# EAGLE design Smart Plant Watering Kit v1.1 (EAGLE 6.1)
COMPANY: ADAFRUIT INDUSTRIES; DRAWN: KTOWN; REV: B
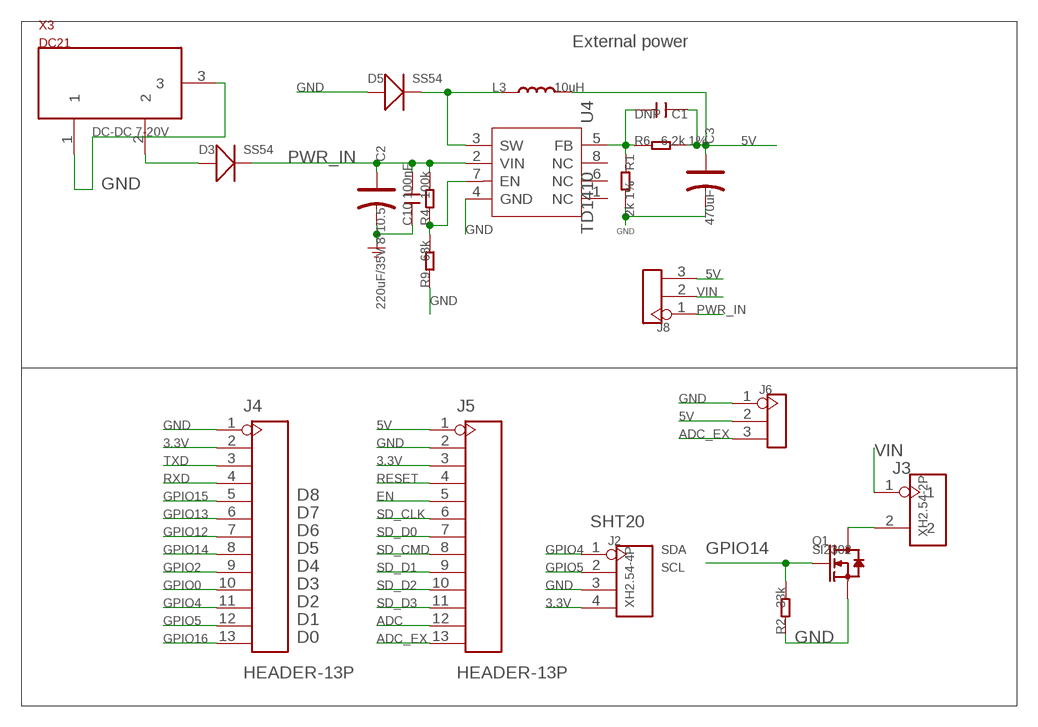
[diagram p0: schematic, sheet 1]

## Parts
C1  DNP  C-0603  [C0603]
C2  220uF/35V 8*10.5  CAP-ELECTRO-E  [ELECTRO-SMD-E-7.8MM]
C3  470uF  CAP-AVX-D  [AVX-D]
C10  100nF  C-0603  [C0603]
D3  SS54  D'SMA'  [D2010]
D5  SS54  D'SMA'  [D2010]
J2  XH2.54-4P  [XH2.54-4P]
J3  XH2.54-2P  [XH2.54-2P]
J4  HEADER-13P  [13P-2.54]
J5  HEADER-13P  [13P-2.54]
J6  HEADER-3P-2.54  [3P-2.54]
J8  HEADER-3P-2.54  [3P-2.54]
L3  10uH  DISCRETE_L0630  [L0630]
Q1  SI2302  MOSFET-N'SOT23'  [SOT23]
R1  2k 1%  R-0603  [R0603]
R2  33k  R-0603  [R0603]
R4  100k  R-0603  [R0603]
R6  6.2k 1%  R-0603  [R0603]
R9  68k  R-0603  [R0603]
U4  TD1410  [SOP8]
X3  DC21  POWERSUPPLY_DC21MMX  [POWERSUPPLY_DC-21MM]

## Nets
3.3V: J2.4 J4.2 J5.3
5V: C1.1 C3.+ J5.1 J6.2 J8.3 L3.2 R6.2
ADC: J5.12
ADC_EX: J5.13 J6.3
EN: J5.5
GND: C2.- C3.- C10.1 D5.+ J2.3 J4.1 J5.2 J6.1 Q1.2(S) R1.2 R2.1 R9.1 U4.4(GND) X3.1 X3.3
GPIO0: J4.10
GPIO2: J4.9
GPIO4: J2.1 J4.11
GPIO5: J2.2 J4.12
GPIO12: J4.7
GPIO13: J4.6
GPIO14: J4.8 Q1.1(G) R2.2
GPIO15: J4.5
GPIO16: J4.13
N$1: D3.+ X3.2
N$4: J3.2 Q1.3(D)
N$12: R4.1 R9.2 U4.7(EN)
N$38: D5.- L3.1 U4.3(SW)
N$47: C1.2 R1.1 R6.1 U4.5(FB)
PWR_IN: C2.+ C10.2 D3.- J8.1 R4.2 U4.2(VIN)
RESET: J5.4
RXD: J4.4
SD_CLK: J5.6
SD_CMD: J5.8
SD_D0: J5.7
SD_D1: J5.9
SD_D2: J5.10
SD_D3: J5.11
TXD: J4.3
VIN: J3.1 J8.2
Unconnected: U4.1(NC) U4.6(NC) U4.8(NC)

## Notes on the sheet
- External power
- DC-DC 7-20V
- D8
- D7
- SHT20
- D6
- D5 | SDA
- D4 | SCL
- D3
- D2
- D1
- D0

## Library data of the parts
C1 C10 = Discrete:C*: Ceramic Capacitors
C2 C3 = Discrete:CAP*: Electrolytic Capacitors,Tantalum Capacitors and Super Capacitors
D3 D5 = Discrete:D*
J2 = Connector:XH2.54-4P
J3 = Connector:XH2.54-2P
J4 J5 = Connector:HEADER-13P
J6 J8 = Connector:HEADER-3P
L3 = L:DISCRETE_L*
Q1 = Discrete:MOSFET-N: IRLL014: http://www.vishay.com/docs/91319/sihll014.pdf
R1 R2 R4 R6 R9 = Discrete:R*
U4 = template:TD1410: 2A 380KHz 20V PWM Buck DC/DC Converter
X3 = SmartPrj:POWERSUPPLY_DC21MM

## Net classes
0 default: width 0.203 mm, drill 0.305 mm, clearance 0.152 mm

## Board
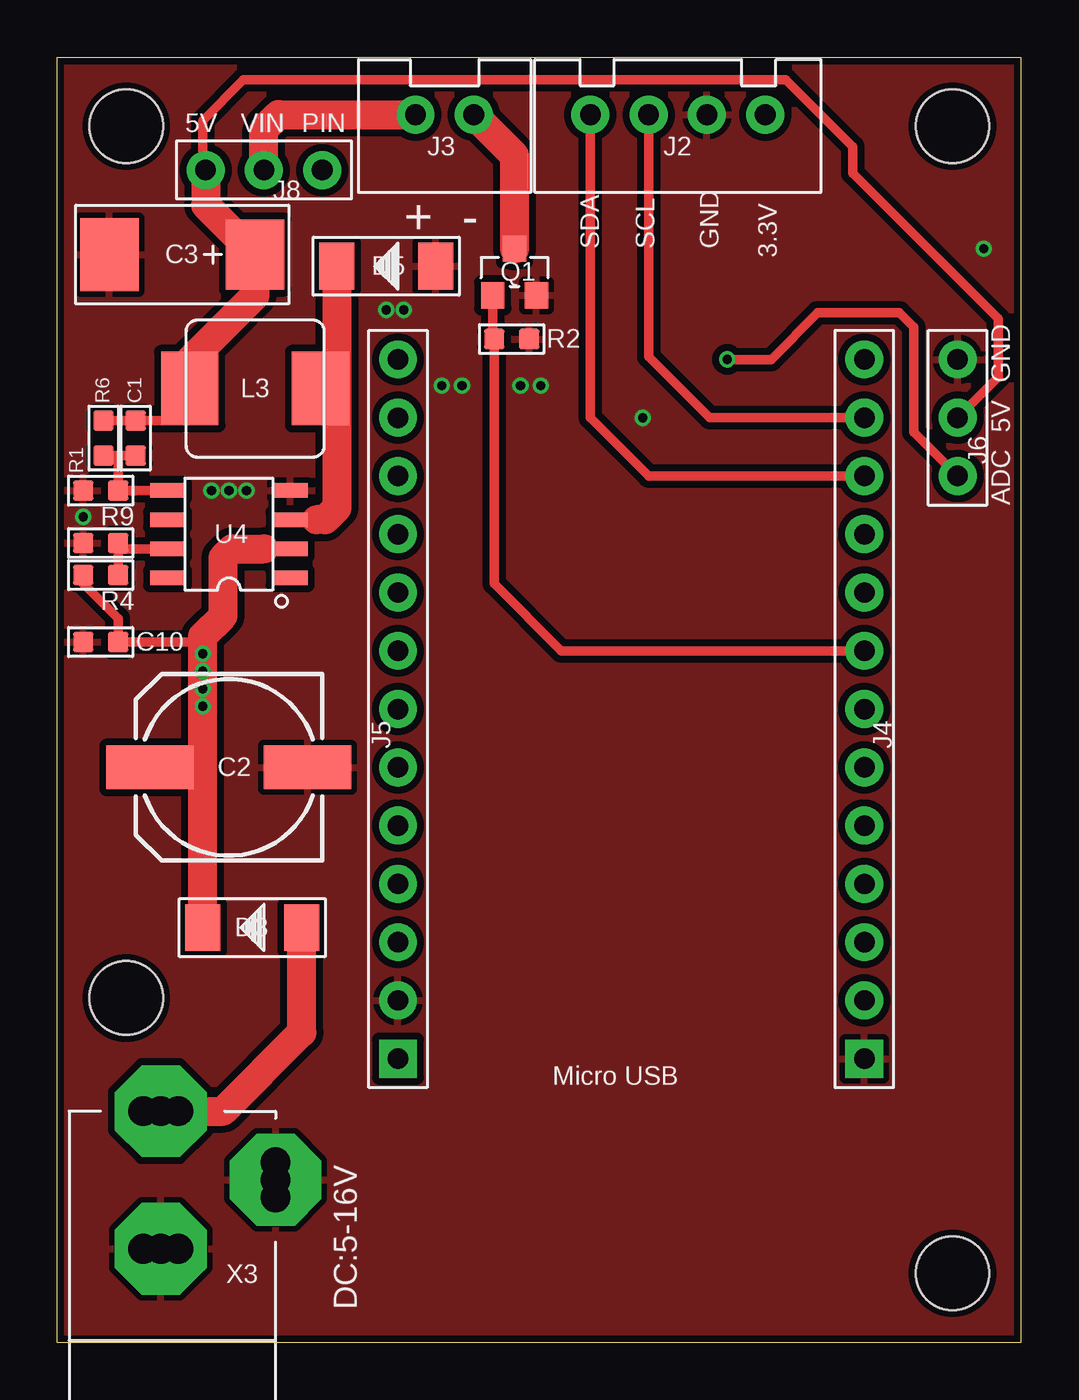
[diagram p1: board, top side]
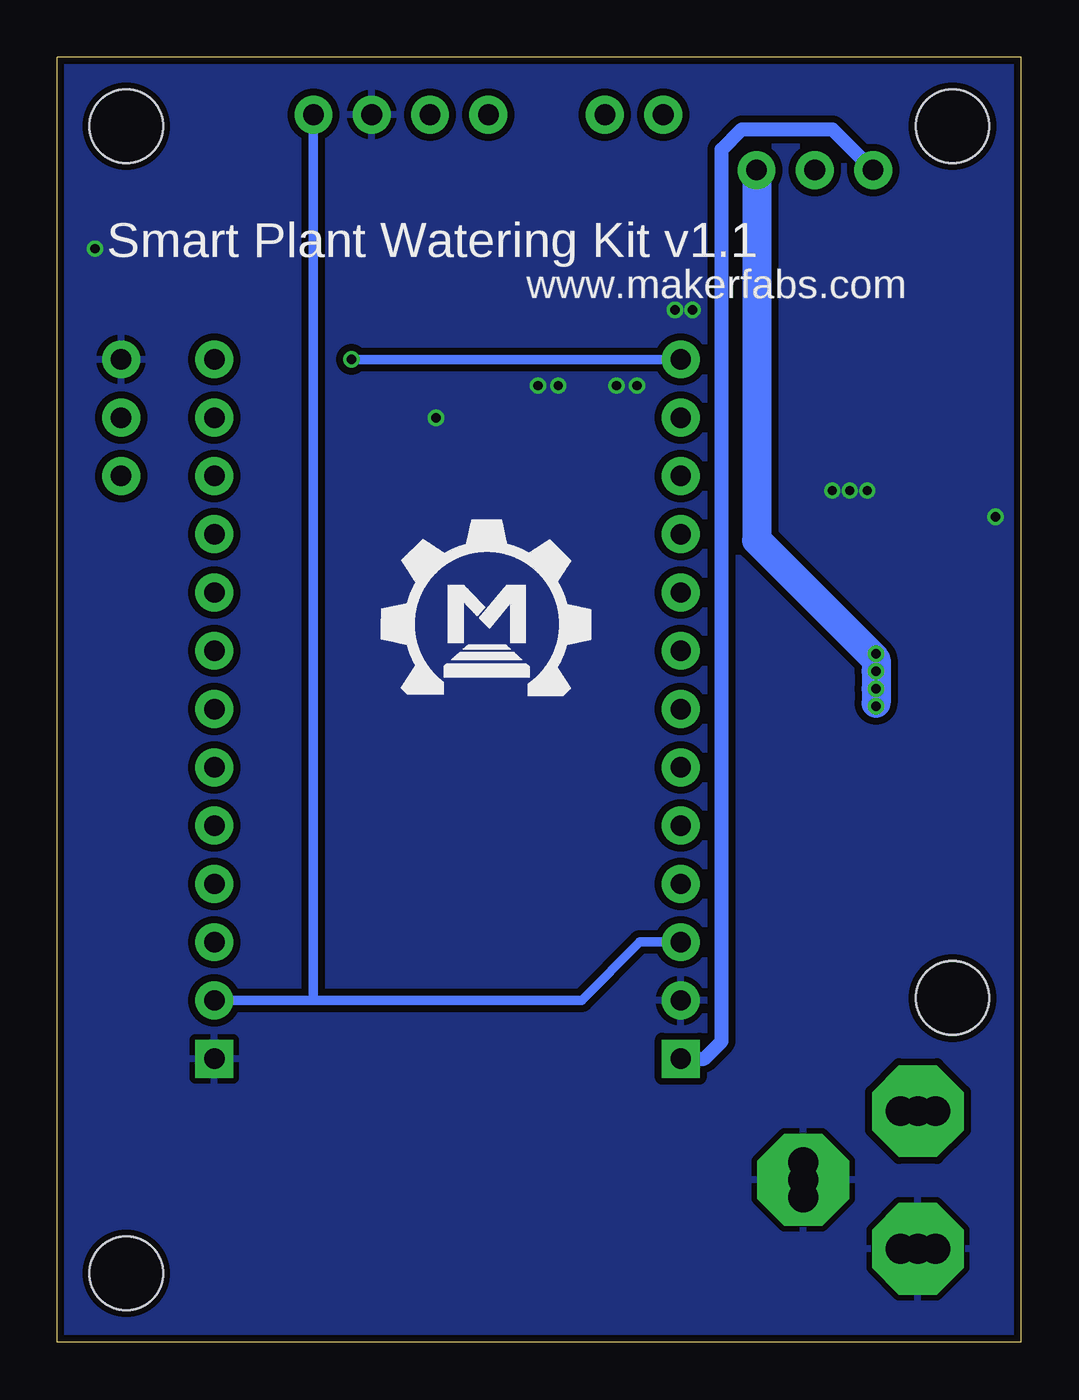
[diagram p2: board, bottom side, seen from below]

Size 42 x 56 mm. Coordinates in mm from the lower left corner, seen from the top.
Outline: 42,0 42,56 0,56 0,0 42,0
Copper layers (1*16): Top 0.035mm / dielectric 1.5mm / Bottom 0.035mm
Design rules: minimum track width 6mil, minimum drill 12mil, track to track 6mil, track to pad 6mil, pad to pad 6mil, via to via 6mil, smd to smd 0mil, copper to edge 10mil, drill to drill 10mil, minimum pad ring 10mil, minimum via ring 6mil, stop-mask expansion 2mil, vias tented up to drill 100mil, thermal gap 10mil
Holes 3.2 mm at 39,3 3,53 39,53 3,15

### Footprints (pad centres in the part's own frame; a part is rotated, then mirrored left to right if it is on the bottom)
C0603 = smd 0.889 x 0.889: 1 -0.762,0; 2 0.762,0
ELECTRO-SMD-E-7.8MM = smd 3.81 x 1.905: + 3.429,0; - -3.429,0
AVX-D = smd 2.54 x 3.048: + -3.175,0 | smd 2.54 x 3.175: - 3.175,0
D2010 = smd 1.524 x 2.032: + -2.159,0; - 2.159,0
XH2.54-4P = drill 0.9 pad 1.651: 1 -3.81,0; 2 -1.27,0; 3 1.27,0; 4 3.81,0
XH2.54-2P = drill 0.9 pad 1.651: 1 -1.27,0; 2 1.27,0
13P-2.54 = drill 0.889 pad 1.651 square: 1 0,15.24 | drill 0.889 pad 1.651: 2 0,12.7; 3 0,10.16; 4 0,7.62; 5 0,5.08; 6 0,2.54; 7 0,0; 8 0,-2.54; 9 0,-5.08; 10 0,-7.62; 11 0,-10.16; 12 0,-12.7; 13 0,-15.24
3P-2.54 = drill 0.9 pad 1.651: 1 0,2.54; 2 0,0; 3 0,-2.54
L0630 = smd 2.5 x 3.2: 1 -2.85,0; 2 2.85,0
SOT23 = smd 1.016 x 1.143: 1 -0.95,-1.016; 2 0.95,-1.016; 3 0,1.016
R0603 = smd 0.889 x 0.889: 1 -0.762,0; 2 0.762,0
SOP8 = smd 0.635 x 1.524: 1 -1.905,-2.667; 2 -0.635,-2.667; 3 0.635,-2.667; 4 1.905,-2.667; 5 1.905,2.667; 6 0.635,2.667; 7 -0.635,2.667; 8 -1.905,2.667
POWERSUPPLY_DC-21MM = drill 1.3 pad 4 octagon: 1 -5.08,-3.353; 2 -0.076,-6.35; 3 -0.076,-0.356 | drill 1.3: 4 -5.08,-4.115; 5 -5.08,-2.591; 6 -0.838,-0.356; 7 0.686,-0.356; 8 -0.838,-6.35; 9 0.686,-6.35

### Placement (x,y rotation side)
C1  3.41,39.41 270 top
C2  7.47,25.05 180 top
C3  5.44,47.41 180 top
C10  1.89,30.52 0 top
D3  8.49,18.07 180 top
D5  14.33,46.9 180 top
J2  27.03,53.5 0 top
J3  16.87,53.5 0 top
J4  35.16,27.59 180 top
J5  14.84,27.59 180 top
J6  39.22,40.29 0 top
J8  9,51.09 270 top
L3  8.62,41.56 180 top
Q1  19.92,46.64 0 top
R1  1.89,37.12 180 top
R2  19.79,43.72 180 top
R4  1.89,33.44 180 top
R6  2.01,39.41 90 top
R9  1.89,34.83 0 top
U4  7.47,35.21 90 top
U$1  [MAKERFABS_0.3]  27.41,28.23 0 bottom
X3  4.43,3.72 180 top

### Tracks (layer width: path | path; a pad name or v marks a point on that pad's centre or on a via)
3.3V
  Bottom 0.406: J2.4 30.84,15.02 30.71,14.89 | J4.2 30.71,14.89 | 30.71,14.89 19.16,14.89 16.62,17.43 J5.3
5V
  Top 0.406: C1.1 R6.2 5.19,40.17 5.95,40.93 5.95,41.38 L3.2 | J8.3 6.33,51.22 6.33,53.25 8.11,55.03 31.73,55.03 34.65,52.11 34.65,50.96 41,44.61 41,42.07 J6.2
  Top 1.27: L3.2 5.77,42.78 8.62,45.63 C3.+ 6.46,49.56 J8.3
  Bottom 0.61: J5.1 13.82,12.35 13.06,13.12 13.06,51.98 12.17,52.87 8.24,52.87 J8.3
ADC_EX  (via drill 0.41)
  Top 0.406: v29.19,42.83 31.1,42.83 33.13,44.87 36.68,44.87 37.32,44.23 37.32,39.66 J6.3
  Bottom 0.406: J5.13 v29.19,42.83
GND  (via drill 0.41)
  other vias: 1.12,35.98 25.51,40.29 20.17,41.69 21.06,41.69 14.33,44.99 15.09,44.99 6.71,37.12 7.47,37.12 8.24,37.12 16.74,41.69 17.63,41.69 40.37,47.66
  pour Top (isolate 0.305): 0,0 42,0 42,56.2 -0.13,55.94
  pour Bottom (isolate 0.305): 42,0 42,56.2 -0.38,55.94 0,0
GPIO4
  Top 0.406: J4.11 25.76,37.75 23.22,40.29 J2.1
GPIO5
  Top 0.406: J4.12 28.43,40.29 25.76,42.96 J2.2
GPIO14
  Top 0.406: J4.8 21.95,30.13 19.03,33.05 R2.2 18.97,43.78 Q1.1
N$1
  Top 1.27: 10.65,18.45 D3.+ 10.65,13.5 7.22,10.07 X3.2
N$4
  Top 1.27: Q1.3 19.92,51.72 J3.2
N$12
  Top 0.406: R4.1 R9.2 2.9,34.58 U4.7
N$38
  Top 0.406: U4.3 11.28,35.85 | L3.1 12.05,41.56 12.17,41.44 | 12.17,41.31 12.05,41.31
  Top 1.27: 12.17,41.18 12.17,36.36 11.66,35.85 11.28,35.85 | D5.- 12.17,41.44 12.17,41.31 12.17,41.18 | L3.1 11.16,41.56 | 11.03,41.56 11.16,41.56 | 11.16,41.56 11.92,40.8 12.05,40.8 12.05,41.31 | 12.17,41.18 11.79,41.56 11.54,41.56
N$47
  Top 0.406: U4.5 R1.1 2.65,38.64 | R6.1 2.65,38.64 | 2.65,38.64 C1.2
PWR_IN  (via drill 0.41)
  Top 0.406: 6.33,30.39 6.2,30.52 C10.2 2.65,31.53 1.12,33.05 R4.2 | U4.2 9,34.58
  Top 1.27: 9,34.58 7.6,34.58 7.22,34.2 7.22,31.66 6.33,30.77 6.33,30.39 v6.33,30.01 v6.33,29.24 v6.33,28.48 v6.33,27.72 6.33,24.93 | D3.- 6.33,24.93 | C2.+ 6.2,25.05 6.33,24.93
  Bottom 1.27: J8.1 11.54,34.96 6.33,29.75 v6.33,29.24 v6.33,28.48 6.33,27.85
VIN
  Top 1.27: J8.2 9,52.87 9.63,53.5 J3.1

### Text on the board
tPlace: 5V | VIN | PIN | + | - | SDA | SCL | GND | 3.3V | GND | 5V | ADC | Micro USB | DC:5-16V
bPlace: Smart Plant Watering Kit v1.1 | www.makerfabs.com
